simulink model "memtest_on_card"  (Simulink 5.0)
settings: Solver=ode45  StartTime=0.0  StopTime=50  RelTol=1e-3
libraries: ADlibrary x1

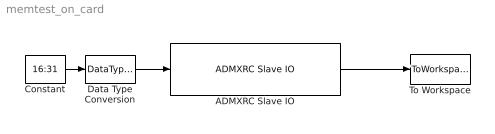
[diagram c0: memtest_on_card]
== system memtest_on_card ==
  ADMXRC Slave IO : ADlibrary/Hardware in the Loop/ADMXRC Slave IO  AncestorBlock=ADlibrary/ADMXRC Simple I//O  filename=e:\tmp3\memtest.bit  clock_freq=33  input_width=16  output_width=16  tll=1000  index=0
  Constant : Constant  Value=16:31
  Data Type Conversion : DataTypeConversion  DataType=uint32
  To Workspace : ToWorkspace  VariableName=simout  SampleTime=-1  SaveFormat=Structure
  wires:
  Constant/1 -> Data Type Conversion/1
  ADMXRC Slave IO/1 -> To Workspace/1
  Data Type Conversion/1 -> ADMXRC Slave IO/1
